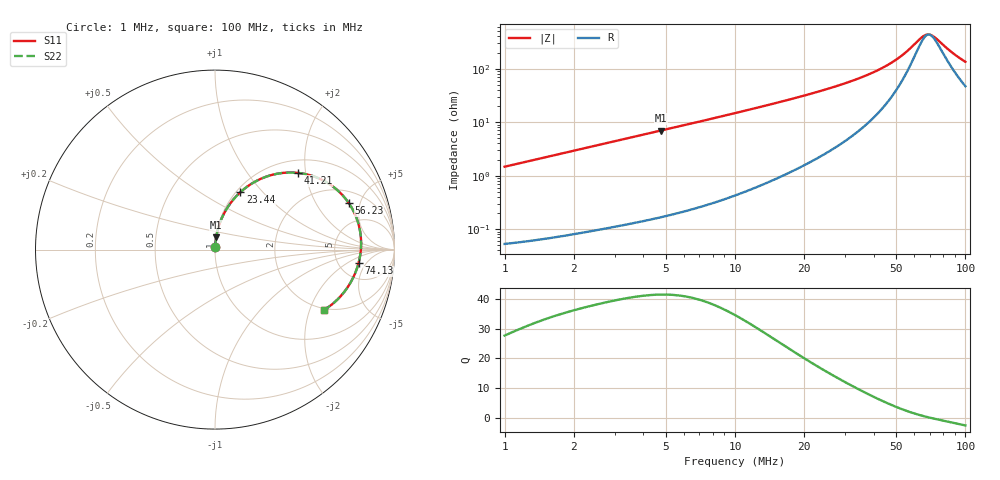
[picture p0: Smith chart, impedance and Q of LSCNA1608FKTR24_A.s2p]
! LSCNA1608FKTR24_A  S-PARAMETER MODEL  ( Standard Model )
! Model Generated by TAIYO YUDEN Corporation (http://www.ty-top.com)
! Version 1.0
! TAIYO YUDEN Control No. 160926
! Copyright(c) 2016 TAIYO YUDEN CO.,LTD. All Rights Reserved.
! Product Description (link to TY-COMPAS)
! https://ds.yuden.co.jp/TYCOMPAS/or/detail?pn=LSCNA1608FKTR24MA&u=M
! Products Name : Inductors
! Characteristics :
!  Inductance : 0.24 [uH] , SRF(min) : - [Hz] , DC Resistance(max) : 50 [mOhm]
!  Rated Current : Saturation  2.3 [A] (dL = 30 [%]), Temp Rise  2.1 [A] (dT = 40 [degC])
!  Case Size : 1.6 x 0.8 / 0.063 x 0.031 [mm/inch] , Thickness : 0.6 / 0.024 [mm/inch]
!  (Conditions: Temperature = 25 [degC] , DC Bias Current = 0 [A])
! External Node Assignments :
!  1  o---GGG---o  2
! GND o---------o GND
! Frequency Range : 1MHz  -  100MHz  [ 402 STEP ]
# MHz S RI R 50
! Freq[MHz].  S11 Real  S11 Imag  S21 Real  S21 Imag  S12 Real  S12 Imag  S22 Real  S22 Imag
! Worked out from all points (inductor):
!   401 points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, 1 MHz to 100 MHz, reference 50 ohm
!   read as one part in series: L = 233 nH near 1.023 MHz
!   highest Q = 41.6 at 4.786 MHz (marker M1), where L = 232 nH
!   self-resonance near 69.64 MHz
!   S11 on the Smith chart (normalised r, x): 1 MHz: 1.00, +0.03; 23.44 MHz: 1.05, +0.76; 41.21 MHz: 1.28, +1.81; 56.23 MHz: 2.87, +3.93; 74.13 MHz: 7.75, -3.29; 100 MHz: 1.94, -2.51
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1  0.000745 0.0147  0.9993 -0.0147  0.9993 -0.0147  0.000745 0.0147
1.62181  0.00126 0.0237  0.9987 -0.0237  0.9987 -0.0237  0.00126 0.0237
2.42661  0.00218 0.0353  0.9978 -0.0353  0.9978 -0.0353  0.00218 0.0353
3.467369  0.00378 0.0503  0.9962 -0.0503  0.9962 -0.0503  0.00378 0.0503
4.786301  0.00648 0.0691  0.9935 -0.0691  0.9935 -0.0691  0.00648 0.0691
6.99842  0.0128 0.1007  0.9872 -0.1007  0.9872 -0.1007  0.0128 0.1007
9.772372  0.0241 0.1399  0.9759 -0.1399  0.9759 -0.1399  0.0241 0.1399
13.33521  0.0445 0.1895  0.9555 -0.1895  0.9555 -0.1895  0.0445 0.1895
17.57924  0.0777 0.2467  0.9223 -0.2467  0.9223 -0.2467  0.0777 0.2467
23.44229  0.1412 0.3196  0.8588 -0.3196  0.8588 -0.3196  0.1412 0.3196
34.27678  0.316 0.4158  0.684 -0.4158  0.684 -0.4158  0.316 0.4158
41.20975  0.461 0.4275  0.539 -0.4275  0.539 -0.4275  0.461 0.4275
45.70882  0.5591 0.4048  0.4409 -0.4048  0.4409 -0.4048  0.5591 0.4048
50.69907  0.6594 0.3497  0.3406 -0.3497  0.3406 -0.3497  0.6594 0.3497
56.23413  0.7459 0.2585  0.2541 -0.2585  0.2541 -0.2585  0.7459 0.2585
63.82635  0.8071 0.1098  0.1929 -0.1098  0.1929 -0.1098  0.8071 0.1098
67.6083  0.8142 0.037  0.1858 -0.037  0.1858 -0.037  0.8142 0.037
70.79458  0.8106 -0.0203  0.1894 0.0203  0.1894 0.0203  0.8106 -0.0203
74.13102  0.7998 -0.0753  0.2002 0.0753  0.2002 0.0753  0.7998 -0.0753
84.13951  0.7396 -0.2088  0.2604 0.2088  0.2604 0.2088  0.7396 -0.2088
92.25714  0.6745 -0.2856  0.3255 0.2856  0.3255 0.2856  0.6745 -0.2856
100  0.6071 -0.3362  0.3929 0.3362  0.3929 0.3362  0.6071 -0.3362
